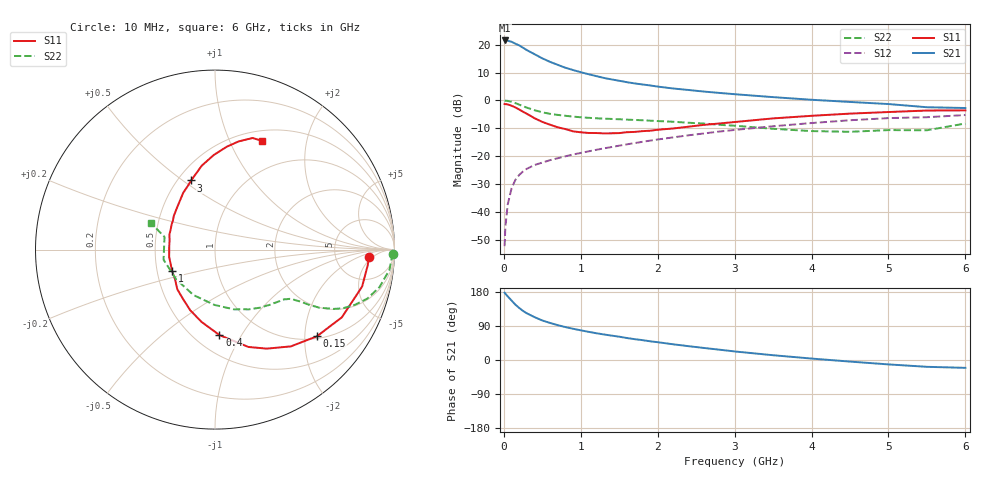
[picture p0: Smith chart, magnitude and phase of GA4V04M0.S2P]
! Infineon Technologies  Discrete & RF Semiconductors
! BF775
! Si NPN RF Bipolar Junction Transistor in SOT23
! VCE = 4 V  IC = 4 mA
! Common Emitter S-Parameters:  May  1996
# GHz  S  MA  R  50
!  f  S11  S21  S12  S22
! GHz  MAG  ANG  MAG  ANG  MAG  ANG  MAG  ANG
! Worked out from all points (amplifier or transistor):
!   36 points, 10 MHz to 6 GHz, reference 50 ohm
!   highest |S21| = 21.5 dB at 10 MHz (marker M1)
!   |S21| within 3 dB of that: start of sweep to 271.7 MHz
!   unconditionally stable (mu >= 1): 888.7 MHz to 3.365 GHz
!   at 250 MHz: K = 0.43, MSG = 22.2 dB, |S12| = -25.5 dB
!   at 1.4 GHz: K = 1.12, MAG = 10.0 dB, |S12| = -16.8 dB
!   at 6 GHz: K = 0.95, MSG = 1.3 dB, |S12| = -5.3 dB
!   S11 on the Smith chart (normalised r, x): 10 MHz: 12, -4; 150 MHz: 1.06, -2.30; 400 MHz: 0.66, -0.81; 1 GHz: 0.60, -0.15; 3 GHz: 0.58, +0.54; 6 GHz: 0.62, +1.33
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0.01  0.8583 -2.9  11.91 177.6  0.0024 89.2  0.9936 -1.3
0.02  0.8554 -5.9  11.68 174.9  0.0053 81.7  0.9855 -2.6
0.05  0.8451 -14.1  11.75 168.0  0.0134 82.8  0.9787 -6.6
0.1  0.8012 -28.1  11.29 157.0  0.0261 75.0  0.9403 -12.8
0.15  0.7453 -40.4  10.41 146.0  0.0373 69.0  0.8919 -17.8
0.2  0.6852 -51.9  9.705 137.3  0.0458 64.8  0.8371 -21.6
0.25  0.6226 -62.4  8.802 129.4  0.0529 60.7  0.7827 -24.7
0.3  0.5733 -71.1  7.971 123.1  0.059 58.7  0.7381 -26.6
0.4  0.477 -87.0  6.732 113.0  0.069 55.4  0.6653 -29.1
0.5  0.4099 -100.5  5.679 104.3  0.0762 54.1  0.609 -30.4
0.6  0.3654 -112.1  4.916 97.8  0.0842 53.8  0.5729 -31.0
0.8  0.3047 -133.6  3.856 86.9  0.0987 53.9  0.5277 -32.2
1  0.2667 -153.9  3.202 78.3  0.1135 54.9  0.4961 -33.6
1.1  0.2595 -162.7  2.952 74.4  0.1211 55.1  0.4856 -34.7
1.3  0.2551 -178.3  2.528 67.4  0.1373 55.5  0.4692 -36.7
1.6  0.2676 161.7  2.119 58.0  0.1621 55.1  0.4507 -40.7
2.2  0.3123 133.3  1.634 41.5  0.2161 52.7  0.4126 -51.4
3  0.4078 109.0  1.29 22.6  0.2939 46.2  0.3503 -72.1
3.5  0.4739 98.9  1.142 12.6  0.3425 40.8  0.3083 -90.5
4.5  0.5775 83.4  0.936 -4.2  0.439 28.2  0.2724 -142.4
5.5  0.656 71.4  0.752 -18.0  0.4975 12.9  0.29 165.9
6  0.6603 66.4  0.728 -20.7  0.5449 8.7  0.3839 157.6
